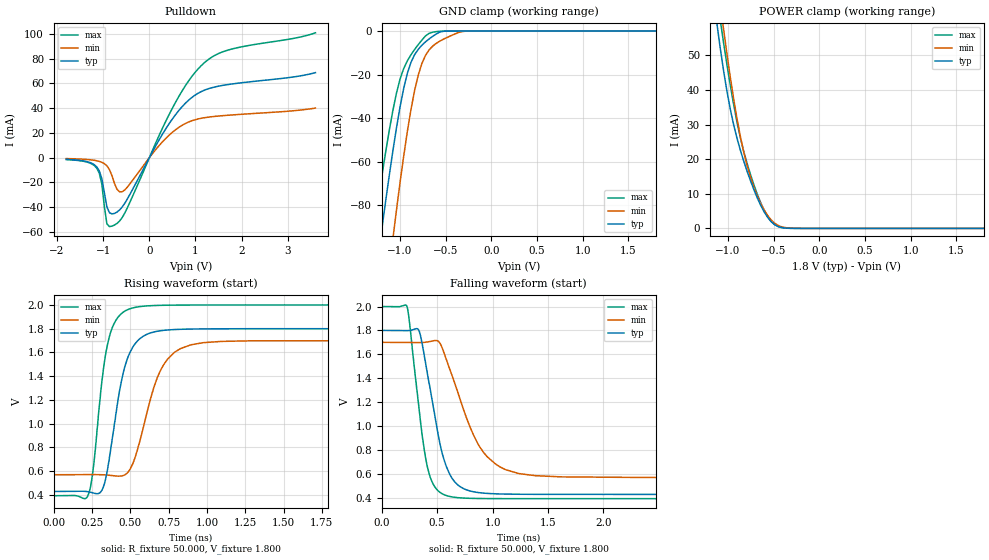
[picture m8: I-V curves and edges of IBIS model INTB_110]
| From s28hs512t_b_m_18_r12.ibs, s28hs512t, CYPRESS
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|   Model INTB_110
[Model] INTB_110
Model_type Open_drain
Polarity   Inverting
Enable   Active-High
Vmeas =  0.900V
Cref =   15.0000pF
Rref =   6.2000k
Vref =   1.8000V
C_comp   5.334pF   5.23pF   5.767pF
[Temperature Range]   25.000   0.125k   -40.000
[Voltage Range]   1.800V   1.700V   2.000V
[Pullup Reference]   1.800V   1.700V   2.000V
[Pulldown Reference]   0.0V   0.0V   0.0V
[POWER Clamp Reference]   1.800V   1.700V   2.000V
[GND Clamp Reference]   0.0V   0.0V   0.0V
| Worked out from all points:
|   slope of the pulldown table from 0 to 0.27 V, typ, clamps not added: 14.9 ohm
|   GND clamp passes 1 mA (typ) near -0.59 V on its own axis
|   POWER clamp passes 1 mA (typ) near -0.48 V on its own axis
|   rising waveform, R_fixture 50.000, V_fixture 1.800: 20-80 % time 113ps typ, 158ps min, 87.3ps max; typ from 0.428 V to 1.8 V
|   falling waveform, R_fixture 50.000, V_fixture 1.800: 20-80 % time 172ps typ, 292ps min, 127ps max; typ from 1.8 V to 0.428 V
[Pulldown]
|Voltage   I(typ)   I(min)   I(max)
-1.8V     -1.334mA   -724.2uA   -1.502mA
-1.14V    -7.446mA   -2.454mA   -8.441mA
-1.03V    -16.88mA   -3.691mA   -21.21mA
-920mV    -39.73mA   -6.551mA   -53.37mA
-755mV    -44.96mA   -20.8mA    -54.34mA
-645mV    -42.15mA   -27.51mA   -51.1mA
-535mV    -36.94mA   -26.09mA   -44.85mA
510mV     31.81mA    20.83mA    40.71mA
840mV     46.04mA    28.63mA    61.36mA
1.17V     54.13mA    32.13mA    75.91mA
1.775V    59.42mA    34.47mA    87.58mA
3.6V      68.65mA    40.07mA    100.8mA
[GND_clamp]
|Voltage   I(typ)   I(min)   I(max)
-1.8V     -294mA     -373mA     -247.3mA
-1.28V    -116.8mA   -168.5mA   -89.46mA
-1.2V     -91.34mA   -138.7mA   -67.04mA
-1.08V    -55.6mA    -96.11mA   -36.91mA
-1.04V    -44.83mA   -82.66mA   -28.74mA
-1V       -34.98mA   -69.76mA   -22.14mA
-920mV    -19.48mA   -46.23mA   -13.73mA
-800mV    -8.377mA   -20.18mA   -6.205mA
-680mV    -3.579mA   -8.59mA    -1.029mA
-560mV    -408.3uA   -4.544mA   -113.8uA
-280mV    -162.8nA   -73.51uA   -82.13nA
1.8V      272.8pA    325nA      188.3pA
[POWER_clamp]
|Voltage   I(typ)   I(min)   I(max)
-1.8V     236.7mA    239.1mA    251.1mA
-1.123V   59.68mA    73.25mA    67.66mA
-1.086V   52.46mA    65.42mA    60.6mA
-1.049V   45.83mA    57.89mA    53.9mA
-938mV    30.03mA    37.57mA    35.87mA
-864mV    22.62mA    26.6mA     26.18mA
-790mV    16.52mA    18.14mA    18.76mA
-716mV    11.21mA    11.92mA    12.63mA
-642mV    6.708mA    7.258mA    7.47mA
-494mV    1.178mA    1.619mA    1.205mA
-272mV    6.291uA    28.11uA    4.439uA
1.8V      0A         0A         0A
[Ramp]
| variable   typ   min   max
dV/dt_r   0.780/0.151n   0.681/0.226n   0.917/0.110n
dV/dt_f   0.823/0.172n   0.678/0.291n   0.965/0.127n
R_load = 50.000
[Rising Waveform]
R_fixture= 50.000
V_fixture= 1.800
V_fixture_min= 1.700
V_fixture_max= 2.000
|time   V(typ)   V(min)   V(max)
0s        428.4mV    569.7mV    392.4mV
221ps     426.8mV    570.6mV    388.3mV
255ps     416.6mV    570.6mV    592.9mV
315ps     440.2mV    569.2mV    1.368V
390ps     939.7mV    560.9mV    1.833V
462ps     1.472V     567.7mV    1.946V
537ps     1.683V     740.2mV    1.981V
717ps     1.786V     1.496V     1.997V
975ps     1.798V     1.682V     1.999V
6ns       1.8V       1.7V       2V
[Falling Waveform]
R_fixture= 50.000
V_fixture= 1.800
V_fixture_min= 1.700
V_fixture_max= 2.000
|time   V(typ)   V(min)   V(max)
0s        1.8V       1.7V       2V
226ps     1.799V     1.699V     2.005V
334ps     1.802V     1.699V     1.167V
383ps     1.594V     1.7V       805.3mV
437ps     1.311V     1.708V     571.9mV
514ps     905.3mV    1.707V     453.9mV
584ps     658.8mV    1.553V     418.4mV
884ps     442.3mV    826mV      394mV
1.236ns   429.7mV    602.8mV    392.8mV
6ns       428.4mV    569.7mV    392.5mV
